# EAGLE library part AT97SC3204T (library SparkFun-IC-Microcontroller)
Atmel Trusted Platform Module 1.2 Datasheet SparkFun Products CryptoCape (DEV-12773) SparkFun CryptoShield (DEV-13183)
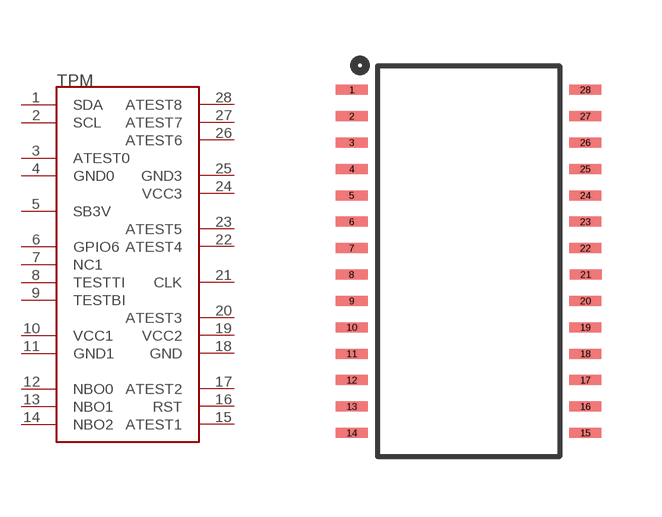
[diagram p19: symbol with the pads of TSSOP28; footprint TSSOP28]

Designator prefix TPM

## AT97SC3204T (PROD_ID: IC-11984; VALUE: ATMEL TPM1.2)  [TSSOP28]
1  SDA
2  SCL
3  ATEST0  pwr
4  GND0  pwr
5  SB3V  pwr
6  GPIO6
7  NC1  nc
8  TESTTI  pwr
9  TESTBI  pwr
10  VCC1  pwr
11  GND1  pwr
12  NBO0  nc
13  NBO1  nc
14  NBO2  nc
15  ATEST1  pwr
16  RST
17  ATEST2  pwr
18  GND  pwr
19  VCC2  pwr
20  ATEST3  pwr
21  CLK
22  ATEST4  pwr
23  ATEST5  pwr
24  VCC3  pwr
25  GND3  pwr
26  ATEST6  pwr
27  ATEST7  pwr
28  ATEST8  pwr

## Footprint TSSOP28 (pad centres in mm)
smd 0.8 x 0.25: 1 -2.921,4.623; 2 -2.921,3.962; 3 -2.921,3.302; 4 -2.921,2.642; 5 -2.921,1.981; 6 -2.921,1.321; 7 -2.921,0.66; 8 -2.927,0; 9 -2.921,-0.66; 10 -2.921,-1.321; 11 -2.921,-1.981; 12 -2.921,-2.642; 13 -2.921,-3.302; 14 -2.921,-3.962; 15 2.921,-3.962; 16 2.921,-3.302; 17 2.921,-2.642; 18 2.921,-1.981; 19 2.921,-1.321; 20 2.921,-0.66; 21 2.927,0; 22 2.921,0.66; 23 2.921,1.321; 24 2.921,1.981; 25 2.921,2.642; 26 2.921,3.302; 27 2.921,3.962; 28 2.921,4.623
